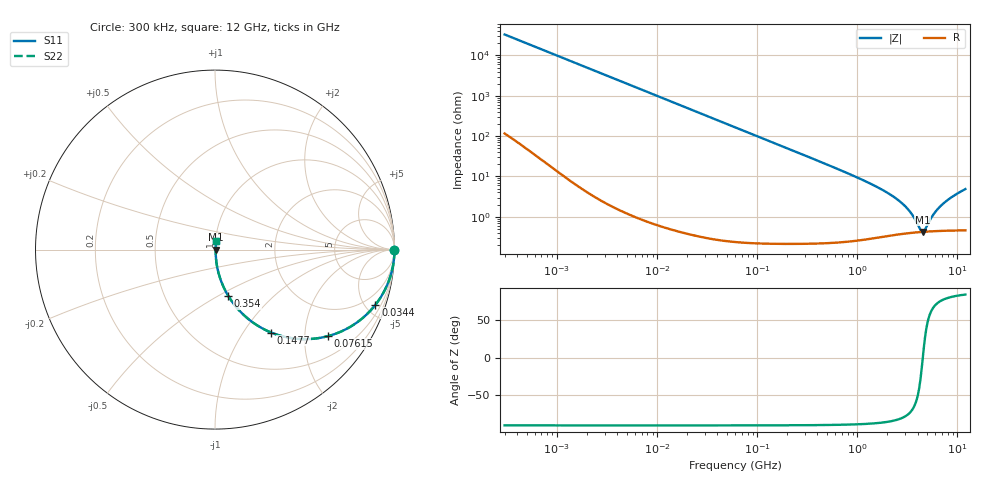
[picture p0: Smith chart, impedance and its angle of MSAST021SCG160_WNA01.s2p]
! MSAST021SCG160_WNA01  S-PARAMETER MODEL  ( Standard Model )
! Model Generated by TAIYO YUDEN Corporation (http://www.ty-top.com)
! Version 1.0
! TAIYO YUDEN Control No. 241126
! Copyright(c) 2024 TAIYO YUDEN CO.,LTD. All Rights Reserved.
! Product Description (link to TY-COMPAS)
! https://ds.yuden.co.jp/TYCOMPAS/or/detail?pn=MSAST021SCG160JWNA01&u=M
! Products Name : Multilayer Ceramic Capacitors
! Characteristics :
!  Capacitance : 16 [pF] , Rated Voltage : 25 [V] , TCC : CG / C0G
!  Case Size : 0.25 x 0.125 / 0.0098 x 0.0049 [mm/inch] , Thickness : 0.125 / 0.0049 [mm/inch]
!  (Conditions: Temperature = 25 [degC] , DC Bias Voltage = 0 [V])
! External Node Assignments :
!  1  o---| |---o  2
! GND o---------o GND
! Frequency Range : 0.3MHz  -  12000MHz  [ 401 STEP ]
# MHZ S RI R 50
! Freq[MHz].  S11 Real  S11 Imag  S21 Real  S21 Imag  S12 Real  S12 Imag  S22 Real  S22 Imag
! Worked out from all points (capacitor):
!   401 points, 300 kHz to 12 GHz, reference 50 ohm
!   read as one part in series: C = 16 pF near 316.3 kHz
!   lowest |Z| = 422 mohm at 4.503 GHz (marker M1)
!   series resonance near 4.503 GHz, so ESL is about 78 pH
!   S11 on the Smith chart (normalised r, x): 300 kHz: open; 34.4 MHz: 1.01, -5.80; 76.15 MHz: 1.00, -2.62; 147.7 MHz: 1.00, -1.35; 354 MHz: 1.00, -0.56; 12 GHz: 1.01, +0.10
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0.3  1 -0.00302  1.97e-05 0.00302  1.97e-05 0.00302  1 -0.00302
1.769972  0.9997 -0.0178  0.000331 0.0178  0.000331 0.0178  0.9997 -0.0178
10.44266  0.9891 -0.1036  0.0109 0.1036  0.0109 0.1036  0.9891 -0.1036
20.79434  0.9582 -0.1998  0.0418 0.1998  0.0418 0.1998  0.9582 -0.1998
34.39878  0.8934 -0.3082  0.1066 0.3082  0.1066 0.3082  0.8934 -0.3082
60  0.7338 -0.4413  0.2662 0.4413  0.2662 0.4413  0.7338 -0.4413
76.15486  0.6312 -0.4816  0.3688 0.4816  0.3688 0.4816  0.6312 -0.4816
104.6549  0.4755 -0.4983  0.5245 0.4983  0.5245 0.4983  0.4755 -0.4983
147.6816  0.3131 -0.4622  0.6869 0.4622  0.6869 0.4622  0.3131 -0.4622
225.6362  0.1637 -0.3676  0.8363 0.3676  0.8363 0.3676  0.1637 -0.3676
353.9943  0.0742 -0.2583  0.9258 0.2583  0.9258 0.2583  0.0742 -0.2583
1048.836  0.0104 -0.0879  0.9896 0.0879  0.9896 0.0879  0.0104 -0.0879
2088.533  0.00469 -0.0363  0.9953 0.0363  0.9953 0.0363  0.00469 -0.0363
3107.553  0.00412 -0.0162  0.9959 0.0162  0.9959 0.0162  0.00412 -0.0162
3547.679  0.0041 -0.0102  0.9959 0.0102  0.9959 0.0102  0.0041 -0.0102
4270.516  0.00417 -0.00224  0.9958 0.00224  0.9958 0.00224  0.00417 -0.00224
4502.883  0.0042 8.9e-07  0.9958 -8.9e-07  0.9958 -8.9e-07  0.0042 8.9e-07
4747.894  0.00425 0.00224  0.9958 -0.00224  0.9958 -0.00224  0.00425 0.00224
5868.704  0.0045 0.0113  0.9955 -0.0113  0.9955 -0.0113  0.0045 0.0113
6879.757  0.00478 0.0184  0.9952 -0.0184  0.9952 -0.0184  0.00478 0.0184
8966.534  0.00551 0.0312  0.9945 -0.0312  0.9945 -0.0312  0.00551 0.0312
12000  0.0069 0.0479  0.9931 -0.0479  0.9931 -0.0479  0.0069 0.0479
